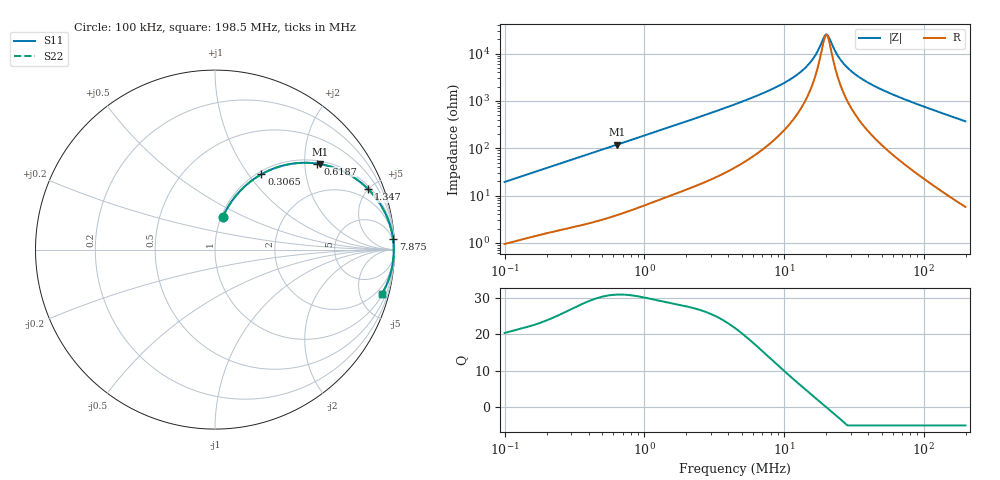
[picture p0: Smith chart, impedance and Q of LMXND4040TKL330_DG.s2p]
! LMXND4040TKL330_DG  S-PARAMETER MODEL  ( General Type )
! Model Generated by TAIYO YUDEN Corporation (http://www.ty-top.com)
! Version 1.0
! TAIYO YUDEN Control No. 191023NI43SB-FBB
! Copyright(c) 2019 TAIYO YUDEN CO.,LTD. All Rights Reserved.
! Product Description (link to TY-COMPAS)
! https://ds.yuden.co.jp/TYCOMPAS/or/detail?pn=LMXND4040TKL330MDG&u=M
! Products Name : Inductors
! Characteristics :
!  Inductance : 33 uH , SRF(min) : 12 MHz , DC Resistance(max) : 0.552 Ohm
!  Rated Current : Saturation :700 mA , Temp Rise : 550 mA
!  Case Size : 4.0 x 4.0 / 0.157 x 0.157 [mm/inch] , Thickness : 1.8 / 0.071 [mm/inch]
!  (Conditions: Temperature = 25 degC , DC Bias Current/Voltage = 0A / 0V)
! External Node Assignments :
!  1  o---GGG---o  2
! GND o---------o GND
! Frequency Range : 0.1MHz  -  198.534594MHz  [ 402 STEP ]
# MHz S RI R 50
! Freq[MHz].  S11 Real  S11 Imag  S21 Real  S21 Imag  S12 Real  S12 Imag  S22 Real  S22 Imag
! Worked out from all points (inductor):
!   401 points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, 100 kHz to 198.5 MHz, reference 50 ohm
!   read as one part in series: L = 30.7 uH near 103.9 kHz
!   highest Q = 30.8 at 642.6 kHz (marker M1), where L = 29.7 uH
!   self-resonance near 19.96 MHz
!   S11 on the Smith chart (normalised r, x): 100 kHz: 1.02, +0.39; 306.5 kHz: 1.04, +1.16; 618.7 kHz: 1.08, +2.31; 1.347 MHz: 1.17, +4.99; 7.875 MHz: 3, +34; 198.5 MHz: 1.12, -7.43
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0.1  0.0446 0.1834  0.9554 -0.1834  0.9554 -0.1834  0.0446 0.1834
0.183581  0.1198 0.3039  0.8802 -0.3039  0.8802 -0.3039  0.1198 0.3039
0.3065  0.2588 0.4199  0.7412 -0.4199  0.7412 -0.4199  0.2588 0.4199
0.356769  0.3172 0.448  0.6828 -0.448  0.6828 -0.448  0.3172 0.448
0.618701  0.5701 0.4791  0.4299 -0.4791  0.4299 -0.4791  0.5701 0.4791
0.642643  0.5878 0.4763  0.4122 -0.4763  0.4122 -0.4763  0.5878 0.4763
1.272844  0.8393 0.3505  0.1607 -0.3505  0.1607 -0.3505  0.8393 0.3505
1.347438  0.8533 0.337  0.1467 -0.337  0.1467 -0.337  0.8533 0.337
2.292754  0.9401 0.2195  0.0599 -0.2195  0.0599 -0.2195  0.9401 0.2195
4.541117  0.9818 0.1125  0.0182 -0.1125  0.0182 -0.1125  0.9818 0.1125
7.875095  0.9922 0.0586  0.00783 -0.0586  0.00783 -0.0586  0.9922 0.0586
12.18657  0.9951 0.0284  0.00487 -0.0284  0.00487 -0.0284  0.9951 0.0284
14.18529  0.9956 0.0194  0.00437 -0.0194  0.00437 -0.0194  0.9956 0.0194
15.89665  0.9959 0.0129  0.00413 -0.0129  0.00413 -0.0129  0.9959 0.0129
17.15079  0.996 0.00868  0.00402 -0.00868  0.00402 -0.00868  0.996 0.00868
19.21992  0.9961 0.00243  0.00393 -0.00243  0.00393 -0.00243  0.9961 0.00243
20.3463  0.9961 -0.000681  0.00391 0.000681  0.00391 0.000681  0.9961 -0.000681
24.59978  0.996 -0.0111  0.00401 0.0111  0.00401 0.0111  0.996 -0.0111
29.18318  0.9957 -0.0208  0.00431 0.0208  0.00431 0.0208  0.9957 -0.0208
38.06772  0.9947 -0.0373  0.00526 0.0373  0.00526 0.0373  0.9947 -0.0373
56.71438  0.9916 -0.0671  0.0084 0.0671  0.0084 0.0671  0.9916 -0.0671
198.5346  0.9291 -0.249  0.0709 0.249  0.0709 0.249  0.9291 -0.249
